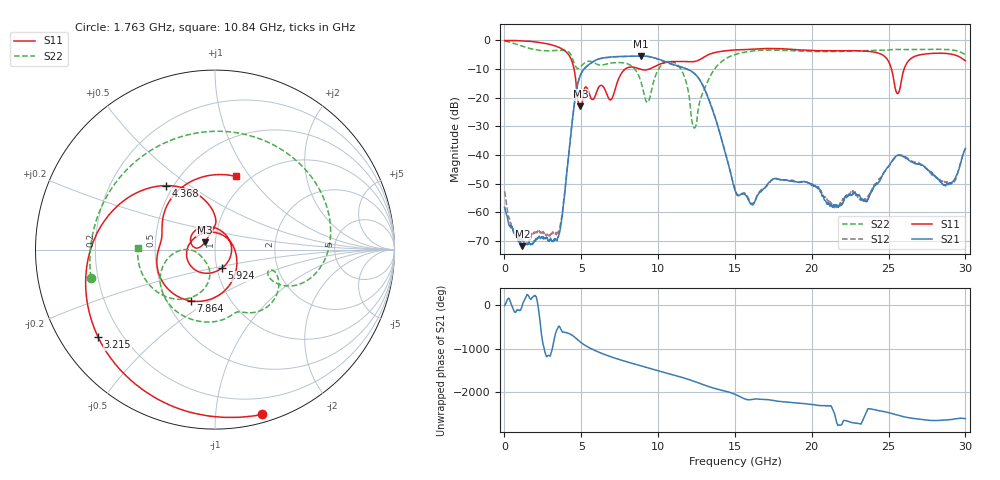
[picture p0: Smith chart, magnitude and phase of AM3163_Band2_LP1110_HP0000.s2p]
!Agilent Technologies,E8364B,MY43040894,A.07.50.67
!Agilent E8364B: A.07.50.67
!Date: Thursday, August 20, 2020 12:02:48
!Correction: S11(Full 2 Port(1,2))
!S21(Full 2 Port(1,2))
!S12(Full 2 Port(1,2))
!S22(Full 2 Port(1,2))
!S2P File: Measurements: S11, S21, S12, S22:
# Hz S  dB  R 50
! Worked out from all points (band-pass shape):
!   3201 points, 10 MHz to 30 GHz, reference 50 ohm
!   highest |S21| = -5.47 dB at 8.885 GHz (marker M1); lowest = -71.8 dB at 1.172 GHz (marker M2)
!   |S21| within 3 dB of the highest: 5.496 GHz to 11.03 GHz (5.533 GHz wide, 67 % of centre)
!   lowest |S11| = -23.1 dB at 4.949 GHz (marker M3), VSWR 1.15, Z = 44.4 + j3.63 ohm
!   |S11| at or under -10 dB: 4.528 GHz to 7.865 GHz (3.337 GHz wide, 53.9 % of centre); 8.799 GHz to 9.439 GHz (639.6 MHz wide, 7.01 % of centre); 25.19 GHz to 26.01 GHz (822.5 MHz wide, 3.21 % of centre)
!   |S22| runs from -30.6 to -0.2 dB; largest |S21 - S12| = 0.01
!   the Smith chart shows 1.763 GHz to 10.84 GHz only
!   S11 on the Smith chart (normalised r, x): 1.763 GHz: 0.06, -1.33; 3.215 GHz: 0.11, -0.33; 4.368 GHz: 0.46, +0.41; 5.924 GHz: 1.05, -0.22; 7.864 GHz: 0.66, -0.42; 10.84 GHz: 0.86, +0.86
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1e7  -0.05 -2.8  -58.33 -6.6  -52.71 6.5  -0.20 -7.5
1.172112e9  -0.16 -48.6  -71.82 20.0  -69.73 -51.2  -2.09 -116.5
1.762541e9  -0.40 -73.9  -71.04 162.0  -67.91 -22.1  -2.99 -167.3
3.215181e9  -1.79 -143.2  -69.90 -99.8  -67.34 -136.4  -3.58 79.6
4.367922e9  -6.98 127.2  -30.41 41.5  -30.39 41.5  -5.54 -20.1
4.948978e9  -23.05 144.8  -12.08 -125.5  -12.08 -125.7  -9.29 -19.7
5.014581e9  -22.69 157.9  -11.33 -143.5  -11.33 -143.7  -8.88 -20.7
5.923653e9  -19.15 -70.1  -6.95 36.5  -6.99 36.4  -8.12 -63.5
6.832725e9  -20.64 80.0  -5.86 -90.9  -5.91 -91.2  -8.03 -86.4
7.863631e9  -10.01 -115.2  -5.60 152.4  -5.62 152.6  -7.95 -127.7
8.885166e9  -10.14 177.4  -5.47 48.1  -5.44 48.1  -14.46 -179.0
1.000979e10  -8.52 130.7  -6.53 -66.3  -6.61 -67.1  -10.24 -118.3
1.084389e10  -7.45 74.2  -8.13 -146.7  -8.35 -146.4  -7.33 178.7
1.236213e10  -7.39 -15.9  -11.55 50.5  -11.60 51.8  -30.58 -91.0
1.5005e10  -3.34 -135.4  -52.39 113.0  -51.99 116.2  -4.95 -145.8
1.784468e10  -2.89 97.6  -48.54 -46.9  -48.43 -45.8  -3.45 78.6
2.000958e10  -3.55 -11.6  -50.60 -118.6  -50.18 -123.7  -3.89 -17.4
2.22682e10  -3.61 -100.5  -54.91 -134.6  -54.14 -134.4  -3.81 -95.9
2.500479e10  -7.42 149.0  -43.95 52.7  -44.06 54.8  -3.35 -169.3
2.559522e10  -18.56 179.2  -40.10 -3.1  -40.19 -1.8  -3.18 174.5
2.875354e10  -4.56 98.1  -50.27 -114.6  -49.53 -114.7  -3.19 90.7
3e10  -7.10 49.9  -37.70 -84.3  -37.84 -86.8  -4.90 53.8
